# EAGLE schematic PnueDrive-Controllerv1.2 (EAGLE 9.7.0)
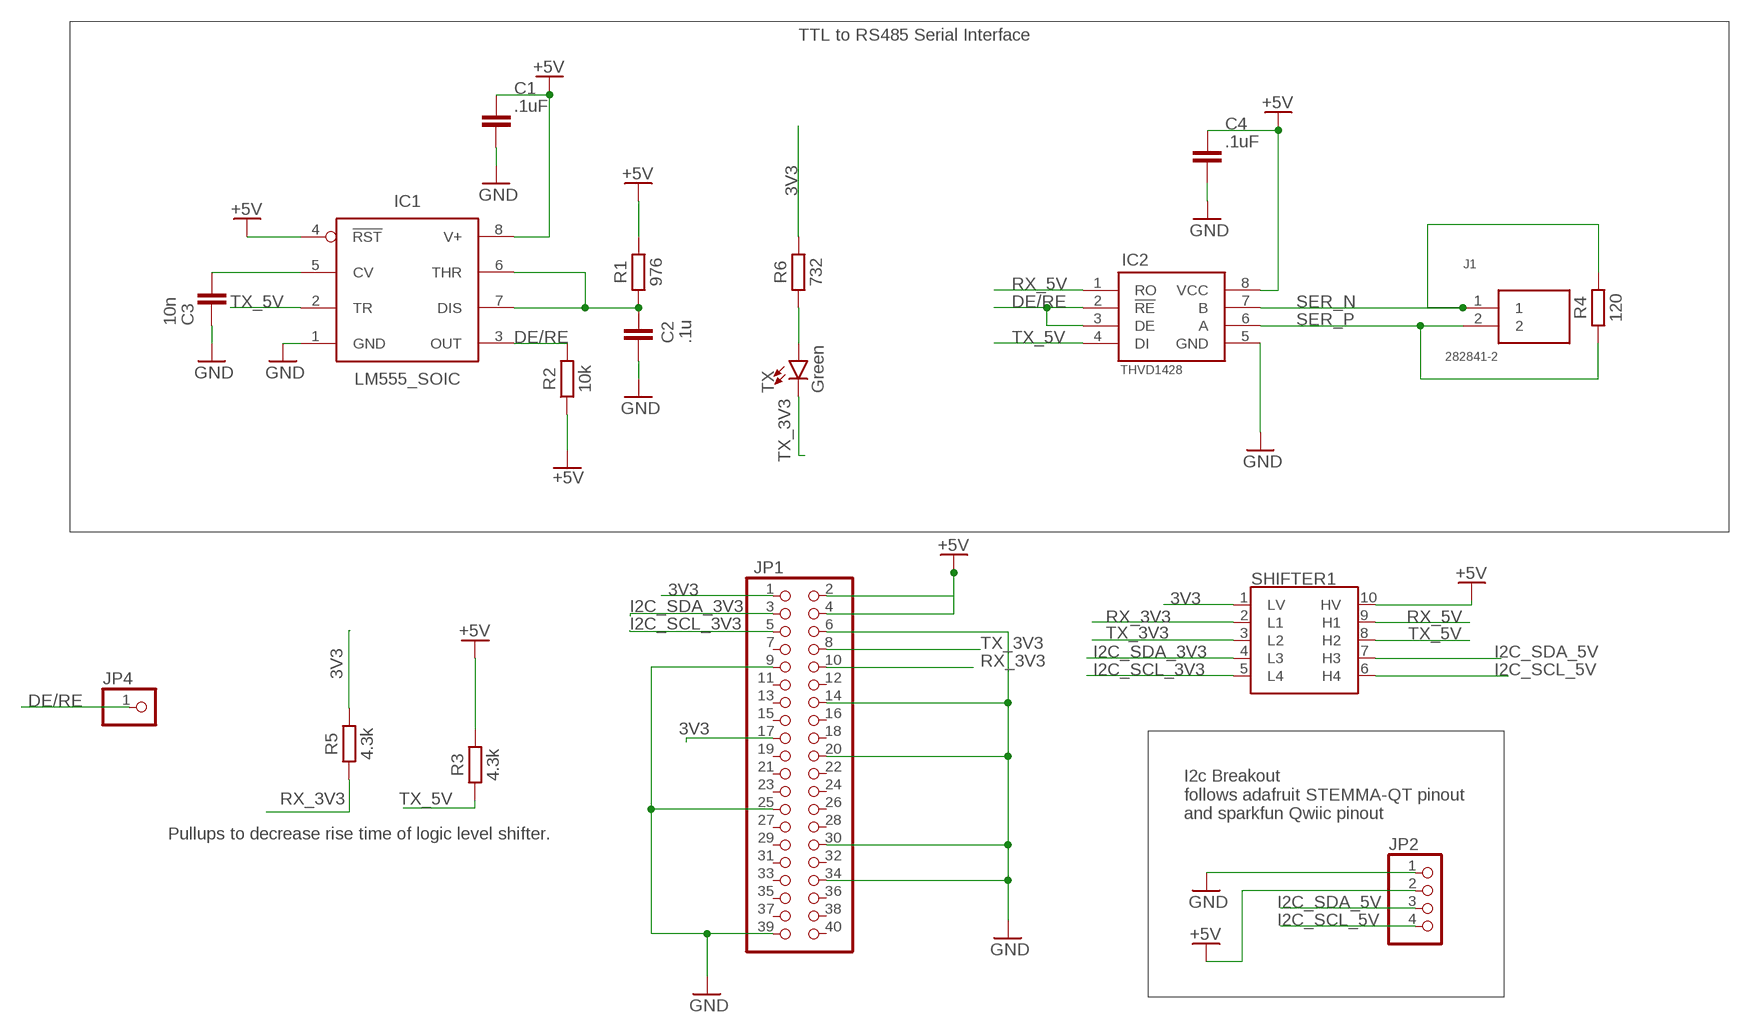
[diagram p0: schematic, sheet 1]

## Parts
C1  .1uF  C_CHIP-0805(2012-METRIC)  [CAPC2012X110]
C2  .1u  C_CHIP-0805(2012-METRIC)  [CAPC2012X110]
C3  10n  C_CHIP-0805(2012-METRIC)  [CAPC2012X110]
C4  .1uF  C_CHIP-0805(2012-METRIC)  [CAPC2012X110]
IC1  LM555_SOIC  [SOIC127P599X175-8N]
IC2  THVD1428  SN65HVD08DR  [SOIC127P600X175-8N]
J1  282841-2  [2828412]
JP1  PINHD-2X20  [2X20]
JP2  PINHD-1X4  [1X04]
JP4  PINHD-1X1  [1X01]
R1  976  R_CHIP-0805(2012-METRIC)  [RESC2012X65]
R2  10k  R_CHIP-0805(2012-METRIC)  [RESC2012X65]
R3  4.3k  R_CHIP-0805(2012-METRIC)  [RESC2012X65]
R4  120  R_CHIP-0805(2012-METRIC)  [RESC2012X65]
R5  4.3k  R_CHIP-0805(2012-METRIC)  [RESC2012X65]
R6  732  R_CHIP-0805(2012-METRIC)  [RESC2012X65]
SHIFTER1  POLOLU_LOGIC_SHIFTERPOLOLU  [POLOLU_LOGIC_SHIFTER]
TX  Green  LED3MM  [LED_3MM]

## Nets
3V3: JP1.1 JP1.17 R5.2 R6.2 SHIFTER1.1(LV)
+5V: C1.1 C4.1 IC1.4(!RST) IC1.8(V+) IC2.8(VCC) JP1.2 JP1.4 JP2.2 R1.2 R2.1 R3.2 SHIFTER1.10(HV)
CV: C3.1 IC1.5(CV)
DE/RE: IC1.3(OUT) IC2.2(!RE) IC2.3(DE) JP4.1 R2.2
GND: C1.2 C2.2 C3.2 C4.2 IC1.1(GND) IC2.5(GND) JP1.6 JP1.9 JP1.14 JP1.20 JP1.25 JP1.30 JP1.34 JP1.39 JP2.1
I2C_SCL_3V3: JP1.5 SHIFTER1.5(L4)
I2C_SCL_5V: JP2.4 SHIFTER1.6(H4)
I2C_SDA_3V3: JP1.3 SHIFTER1.4(L3)
I2C_SDA_5V: JP2.3 SHIFTER1.7(H3)
N$1: R6.1 TX.A
RX_3V3: JP1.10 R5.1 SHIFTER1.2(L1)
RX_5V: IC2.1(RO) SHIFTER1.9(H1)
SER_N [impedance_120]: IC2.7(B) J1.1 R4.2
SER_P [impedance_120]: IC2.6(A) J1.2 R4.1
THRESH: C2.1 IC1.6(THR) IC1.7(DIS) R1.1
TX_3V3: JP1.8 SHIFTER1.3(L2) TX.K(C)
TX_5V: IC1.2(TR) IC2.4(DI) R3.1 SHIFTER1.8(H2)
Unconnected: JP1.7 JP1.11 JP1.12 JP1.13 JP1.15 JP1.16 JP1.18 JP1.19 JP1.21 JP1.22 JP1.23 JP1.24 JP1.26 JP1.27 JP1.28 JP1.29 JP1.31 JP1.32 JP1.33 JP1.35 JP1.36 JP1.37 JP1.38 JP1.40

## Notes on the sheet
- TTL to RS485 Serial Interface
- I2c Breakout
  follows adafruit STEMMA-QT pinout
  and sparkfun Qwiic pinout
- Pullups to decrease rise time of logic level shifter.

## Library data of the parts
C1-C4 = Capacitor:C: Capacitor - Generic; CATEGORY: Capacitor
IC1 = IC_Clock-Timing:*555: TIMER 555 General purpose precision timers NE555 : Texas Datasheet, Diodes Incorporated Datasheet LM555 Datasheet LMC555 Datasheet ICM7555 : Maxim Integrated Datasheet, Renesas Electronics America Inc Datasheet; CATEGORY: IC_Clock-Timing; CURRENT-SUPPLY: 10mA; DESCRIPTION: IC OSC SGL TIMER 100KHZ 8-SOIC; FREQUENCY: 100kHz; MANUFACTURER: Texas Instruments; MPN: LM555CM/NOPB; OPERATING_TEMP: 0°C to 70°C; PART_STATUS: Active; ROHS_COMPLIANT: ROHS3 Compliant; SUB-CATEGORY: Timer
IC2 = Library:SN65HVD08DR: RS-422/RS-485 Interface IC Low-Power, Slew-Rate-Limited RS-485/RS-422 Transceivers Source: Datasheet; DESCRIPTION: RS-485 Interface IC; HEIGHT: 1.75mm; MANUFACTURER_NAME: Texas Instruments; MANUFACTURER_PART_NUMBER: SN65HVD08DR; MOUSER_PART_NUMBER: 595-SN65HVD08DR; MOUSER_PRICE-STOCK: https://www.mouser.com/ProductDetail/Texas-Instruments/SN65HVD08DR?qs=QViXGNcIEAtwhwZ8YvgaIA%3D%3D
J1 = Library:282841-2: TERMI-BLOK PCB MOUNT 2P. 5; DESCRIPTION: TERMI-BLOK PCB MOUNT 2P. 5; HEIGHT: 15.45mm; MANUFACTURER_NAME: TE Connectivity; MANUFACTURER_PART_NUMBER: 282841-2; MOUSER_PART_NUMBER: 571-2828412; MOUSER_PRICE-STOCK: https://www.mouser.co.uk/ProductDetail/TE-Connectivity/282841-2?qs=gdajpSf3VLd4K34xU%252BwLgw%3D%3D
JP1 = pinhead:PINHD-2X20: PIN HEADER
JP2 = pinhead:PINHD-1X4: PIN HEADER
JP4 = pinhead:PINHD-1X1: PIN HEADER
R1-R6 = Resistor:R: Resistor Fixed - Generic; CATEGORY: Resistor; SUB-CATEGORY: Fixed
SHIFTER1 = Library:POLOLU_LOGIC_SHIFTER: Logic Level Shifter, 4-Channel, Bidirectional Pololu Link This tiny logic level shifter features four bi-directional channels, allowing for safe and easy communication between devices operating at different logic levels. It can convert signals as low as 1.5 V to as high as 18 V and vice versa, and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
TX = SparkFun-LED:LED: LED (Generic); PROD_ID: DIO-08794

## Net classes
2 impedance_120: width 0.117 mm, clearance 0.203 mm to class 0, clearance 0.203 mm to class 1

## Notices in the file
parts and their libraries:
SparkFun-LED: Licensing: Creative Commons ShareAlike 4.0 International - https://creativecommons.org/licenses/by-sa/4.0
